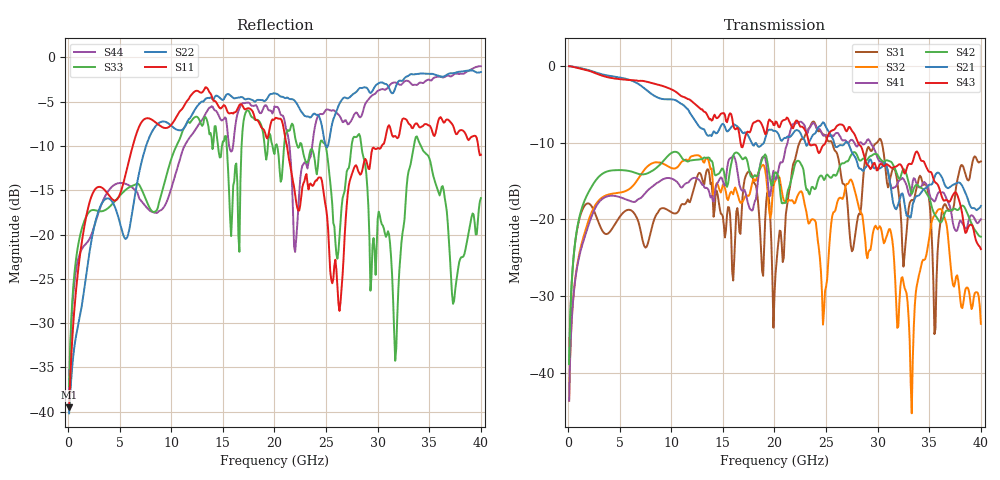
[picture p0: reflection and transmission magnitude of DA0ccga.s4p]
! ADC12DJ3200QML-SP
! 196-pin NWE package
! CCGA Ceramic Package with columns (ceramic column grid array)
! Texas Instruments 4/21/2021
! Single-ended  S-parameters
! PORT#  PORT_NAME  NET_NAME
! PORT1:  DAxN.DIEBUMP DAxN
! PORT2:  DAxN.BGA  DAxN
! PORT3:  DAxP.DIEBUMP DAxP
! PORT4:  DAxP.BGA  DAxP
! Touchstone Ver. 1.0
! Number of ports is 4
# Hz	S	MA	R	50.000000
! SCATTERING PARAMETERS  :
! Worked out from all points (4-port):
!   400 points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, 100 MHz to 40 GHz, reference 50 ohm
!   strongest paths, dB at 100 MHz, 10.1 GHz, 20.1 GHz, 30.1 GHz, 40 GHz:
!     S43: -0.1, -3.1, -7.3, -13.2, -23.9
!     S21: -0.1, -4.4, -8.5, -13.4, -18.2
!     S42: -38.8, -11.3, -13.9, -11.8, -22.2
!     S41: -43.6, -14.7, -14.8, -12.3, -20.0
!     S32: -43.6, -13.4, -14.9, -21.1, -33.6
!     S31: -38.8, -19.1, -27.1, -9.7, -12.5
!   lowest |S11| = -39.5 dB at 100 MHz (marker M1), VSWR 1.02, Z = 51 + j0.465 ohm
!   |S11| at or under -10 dB: start of sweep to 6.268 GHz; 21.21 GHz to 30.39 GHz (9.18 GHz wide, 35.6 % of centre); 39.74 GHz to end of sweep
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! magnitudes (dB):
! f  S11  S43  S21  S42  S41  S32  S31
! 100 MHz  -39.5  -0.1  -0.1  -38.8  -43.6  -43.6  -38.8
! 8.4 GHz  -7.3  -2.4  -4.0  -13.5  -15.5  -12.6  -19.8
! 27.4 GHz  -13.5  -8.2  -11.0  -11.7  -9.7  -14.8  -23.4
! 31.7 GHz  -8.9  -13.2  -18.6  -13.5  -15.8  -27.9  -13.7
! 33.3 GHz  -8.0  -12.8  -19.0  -16.7  -16.0  -45.2  -17.5
! 35.5 GHz  -8.9  -15.0  -14.5  -19.3  -17.7  -19.5  -34.9
! 40 GHz  -11.0  -23.9  -18.2  -22.2  -20.0  -33.6  -12.5
